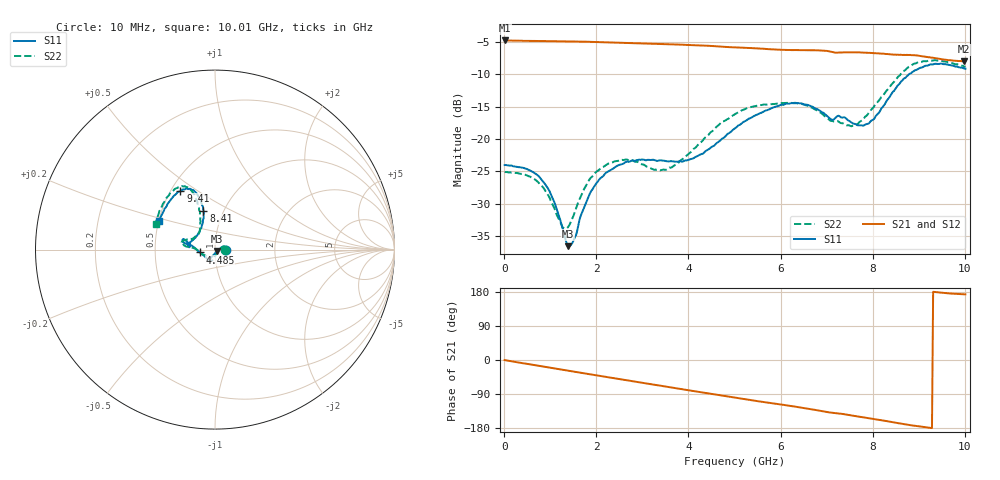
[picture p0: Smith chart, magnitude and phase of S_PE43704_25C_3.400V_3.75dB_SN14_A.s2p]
! Device ID: PE43704
! Dir: z:\PE43704\PE43704_Char_1_20130516\PE43704\AMB\3p400V\3p75dB
! Serial: 14
! Insertion: A
! Impedance: 50 ohm
! Temp: Amb
! VDD: 3.400V
! Attenuation Step: 3.75dB
! IDD: 1.141219e-01mA
#  Hz  S  RI  R  50
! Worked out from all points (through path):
!   401 points, 10 MHz to 10.01 GHz, reference 50 ohm
!   highest |S21| = -4.80 dB at 10 MHz (marker M1); lowest = -8.0 dB at 9.985 GHz (marker M2)
!   group delay of S21, straight-line fit = 53.1 ps
!   lowest |S11| = -36.5 dB at 1.385 GHz (marker M3), VSWR 1.03, Z = 51.3 - j0.811 ohm
!   |S11| at or under -10 dB: start of sweep to 8.786 GHz
!   |S22| runs from -33.8 to -7.8 dB; largest |S21 - S12| = 0.0041
!   S11 on the Smith chart (normalised r, x): 10 MHz: 1.13, +0.00; 4.485 GHz: 0.84, -0.03; 8.41 GHz: 0.81, +0.36; 9.41 GHz: 0.56, +0.43; 10.01 GHz: 0.50, +0.18
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1e7  0.0629 0.000208  0.5753 -0.00227  0.5756 -0.00223  0.0556 0.000199
8.1e8  0.0453 0.0177  0.546 -0.1615  0.5461 -0.1613  0.0415 0.0136
1.06e9  0.0328 0.00996  0.5292 -0.2083  0.5293 -0.208  0.0305 0.00385
1.26e9  0.021 -0.000147  0.5117 -0.2449  0.5117 -0.2446  0.0198 -0.00726
1.385e9  0.0126 -0.00791  0.4995 -0.2663  0.4994 -0.2664  0.0136 -0.0158
1.51e9  0.00585 -0.0155  0.4862 -0.2877  0.4864 -0.2874  0.00786 -0.0246
1.685e9  -0.00443 -0.0264  0.4664 -0.3163  0.4665 -0.3161  -0.000378 -0.0375
1.935e9  -0.0159 -0.0389  0.4347 -0.3539  0.435 -0.3538  -0.00897 -0.0517
2.26e9  -0.0264 -0.0497  0.3892 -0.3979  0.3894 -0.3976  -0.0175 -0.0622
3.36e9  -0.0402 -0.0553  0.2094 -0.4989  0.21 -0.4987  -0.033 -0.047
4.485e9  -0.0843 -0.0161  0.00529 -0.5218  0.00592 -0.5224  -0.1129 0.00551
5.01e9  -0.1199 0.0149  -0.0824 -0.5022  -0.0821 -0.5025  -0.1547 0.0162
5.985e9  -0.1731 0.057  -0.2224 -0.4347  -0.2202 -0.435  -0.1851 0.0381
6.685e9  -0.1737 0.0387  -0.3135 -0.3679  -0.3138 -0.3677  -0.1654 0.0537
7.585e9  -0.1174 0.0586  -0.3925 -0.2529  -0.392 -0.2525  -0.0902 0.0906
7.935e9  -0.0841 0.1048  -0.4151 -0.2019  -0.4155 -0.2029  -0.0821 0.141
8.36e9  -0.0631 0.2001  -0.4293 -0.1355  -0.429 -0.1371  -0.089 0.2334
8.41e9  -0.0644 0.2143  -0.4304 -0.1274  -0.4303 -0.1288  -0.0949 0.2464
8.86e9  -0.1024 0.3123  -0.4398 -0.0564  -0.437 -0.0581  -0.1479 0.3438
9.41e9  -0.1923 0.3261  -0.4172 0.00997  -0.4171 0.0109  -0.2338 0.3272
9.985e9  -0.3051 0.1686  -0.3942 0.0461  -0.3953 0.0475  -0.3266 0.1535
1.001e10  -0.3107 0.1574  -0.3952 0.0467  -0.3973 0.0478  -0.3297 0.1443
